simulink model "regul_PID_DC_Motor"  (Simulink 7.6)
settings: Solver=ode23t  StartTime=0.0  StopTime=25.0  RelTol=1e-3
InitFcn:
  | clear all
  | close all
  | C1=500;
  | C2=-500;
StopFcn:
  | clc
  | close all, clc
  | load regul_vitesse.mat
  | plot(x(1,:),x(2,:),x(1,:),x(3,:))
  | xlabel('temps')
  | title('Vitesse angulaire et consigne')
  | grid
  | 
  | load Ia_CdePID.mat
  | figure
  | plotyy(y(1,:),y(2,:),y(1,:),y(3,:))
  | xlabel('temps')
  | title('Courant armatures et commande PID')
  | grid
  | 
  | delete *.mat
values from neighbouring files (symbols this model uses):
  A = [1+j -(1-j);1 -2/(1-j)]    [systeme_AX_B_phaseurs.m]
  N = 50;')    [Prog_callbacks.m]    (also in _startup.m = 0.001'))
undefined symbols (not defined in the file or in its folder): constant, Torque
libraries: powerlib x6, powerlib_extras x1

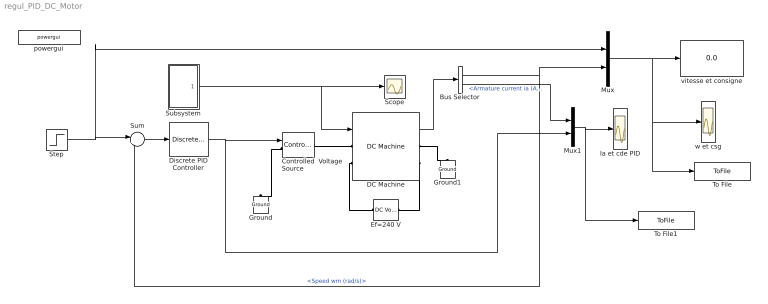
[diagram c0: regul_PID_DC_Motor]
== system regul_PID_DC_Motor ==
  Bus Selector : BusSelector  OutputSignals=Speed wm (rad/s),Armature current ia (A)
  Controlled  Voltage Source : powerlib/Electrical Sources/Controlled Voltage Source  DialogController=POWERSYS.PowerSysDialog  SystemSampleTime=-1  Initialize=on  Source_Type=AC  Amplitude=0  Phase=0  Frequency=0  Measurements=None
  DC Machine : powerlib/Machines/DC Machine  DialogController=POWERSYS.PowerSysDialog  SystemSampleTime=-1  PresetModel=No  MechanicalLoad=Torque TL  FieldType=Wound  ShowDetailedParameters=on  RLa="[ 0.6  0.012]"  RLf="[ 240  120]"  Laf=1.8  MachineConstant=Torque constant (N.m/A)  Ke=1.8  Kt=1.8  J=1  Bm=0  Tf=0  w0=1  Ifinit=1  TsPowergui=0  TsBlock=-1
  Discrete PID Controller : powerlib_extras/Discrete  Control Blocks/Discrete PID Controller  DialogController=POWERSYS.PowerSysDialog  SystemSampleTime=-1  Kp=0.5  Ki=5  Kd=1  TcD=1  Par_Limits=[500 -500]  Init=0  Ts=0.1
  Ef=240 V : powerlib/Electrical Sources/DC Voltage Source  Description=source block  DialogController=POWERSYS.PowerSysDialog  SystemSampleTime=-1  Amplitude=240  Measurements=None
  Ground : powerlib/Elements/Ground  DialogController=POWERSYS.PowerSysDialog  PhysicalDomain=powersysdomain  SubClassName=unknown  LeftPortType=p1  RightPortType=p1  LConnTagsString=a
  Ground1 : powerlib/Elements/Ground  DialogController=POWERSYS.PowerSysDialog  PhysicalDomain=powersysdomain  SubClassName=unknown  LeftPortType=p1  RightPortType=p1  LConnTagsString=a
  Ia et cde PID : Scope
  Mux : Mux  Inputs=2
  Mux1 : Mux  Inputs=2
  Scope : Scope
  Step : Step  Time=0  After=100  SampleTime=0
  Subsystem : Subsystem
  Sum : Sum  Inputs=|+-
  To File : ToFile  Filename=regul_vitesse  MatrixName=x
  To File1 : ToFile  Filename=Ia_CdePID  MatrixName=y
  powergui : powerlib/powergui  Priority=2  SystemSampleTime=-1  SimulationMode=Continuous  SampleTime=0  frequency=60  SPID=off  DisableSnubberDevices=off  DisableRonSwitches=off  DisableVfSwitches=off  SwTol=0  Interpol=off  frequencyindice=0  echomessages=off  HookPort=off  DisplayEquations=off  FunctionMessages=off  EnableUseOfTLC=off  x0status=blocks  RestoreLinks=warning  ResistiveCurrentMeasurement=off  Frange=logspace(0,3,50)  Ylog=off  Xlog=off  ShowGrid=off  save=off  variable=ZData  ZoomFFT=on  StartTime=0.0  cycles=1  DisplayStyle=off  fundamental=60  FreqAxis=off  MaxFrequency=1000  frequencyindicesteady=1  RmsSteady=1  display=off  Ts=0  methode=off
  vitesse et consigne : Display
  w et csg : Scope
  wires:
  Discrete PID Controller/1 -> Controlled  Voltage Source/1, Mux1/2
  Subsystem/1(Perturb) -> DC Machine/1, Scope/1
  DC Machine/1 -> Bus Selector/1
  Step/1 -> Mux/1, Sum/1
  Mux/1 -> vitesse et consigne/1, To File/1, w et csg/1
  Mux1/1 -> Ia et cde PID/1, To File1/1
  Sum/1 -> Discrete PID Controller/1
  Bus Selector/1 -> Mux/2, Sum/2  "<Speed wm (rad/s)>"
  Bus Selector/2 -> Mux1/1  "<Armature current ia (A)>"
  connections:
  Controlled  Voltage Source/RConn1 -- DC Machine/LConn1
  Controlled  Voltage Source/LConn1 -- Ground/LConn1
  DC Machine/RConn1 -- Ground1/LConn1
  Ef=240 V/LConn1 -- DC Machine/RConn2
  Ef=240 V/RConn1 -- DC Machine/LConn2

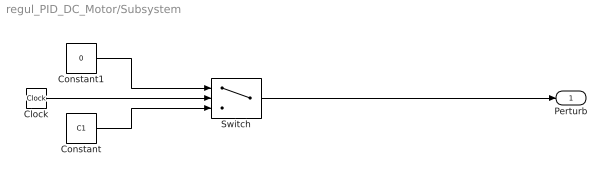
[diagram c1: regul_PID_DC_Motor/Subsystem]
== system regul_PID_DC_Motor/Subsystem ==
  Clock : Clock
  Constant : Constant  Value=C1
  Constant1 : Constant  Value=0
  Switch : Switch  Threshold=10
  Perturb : Outport
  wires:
  Clock/1 -> Switch/2
  Constant1/1 -> Switch/1
  Constant/1 -> Switch/3
  Switch/1 -> Perturb/1
